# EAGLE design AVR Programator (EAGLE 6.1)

## Sheet 1 of 3: Atmel programmer
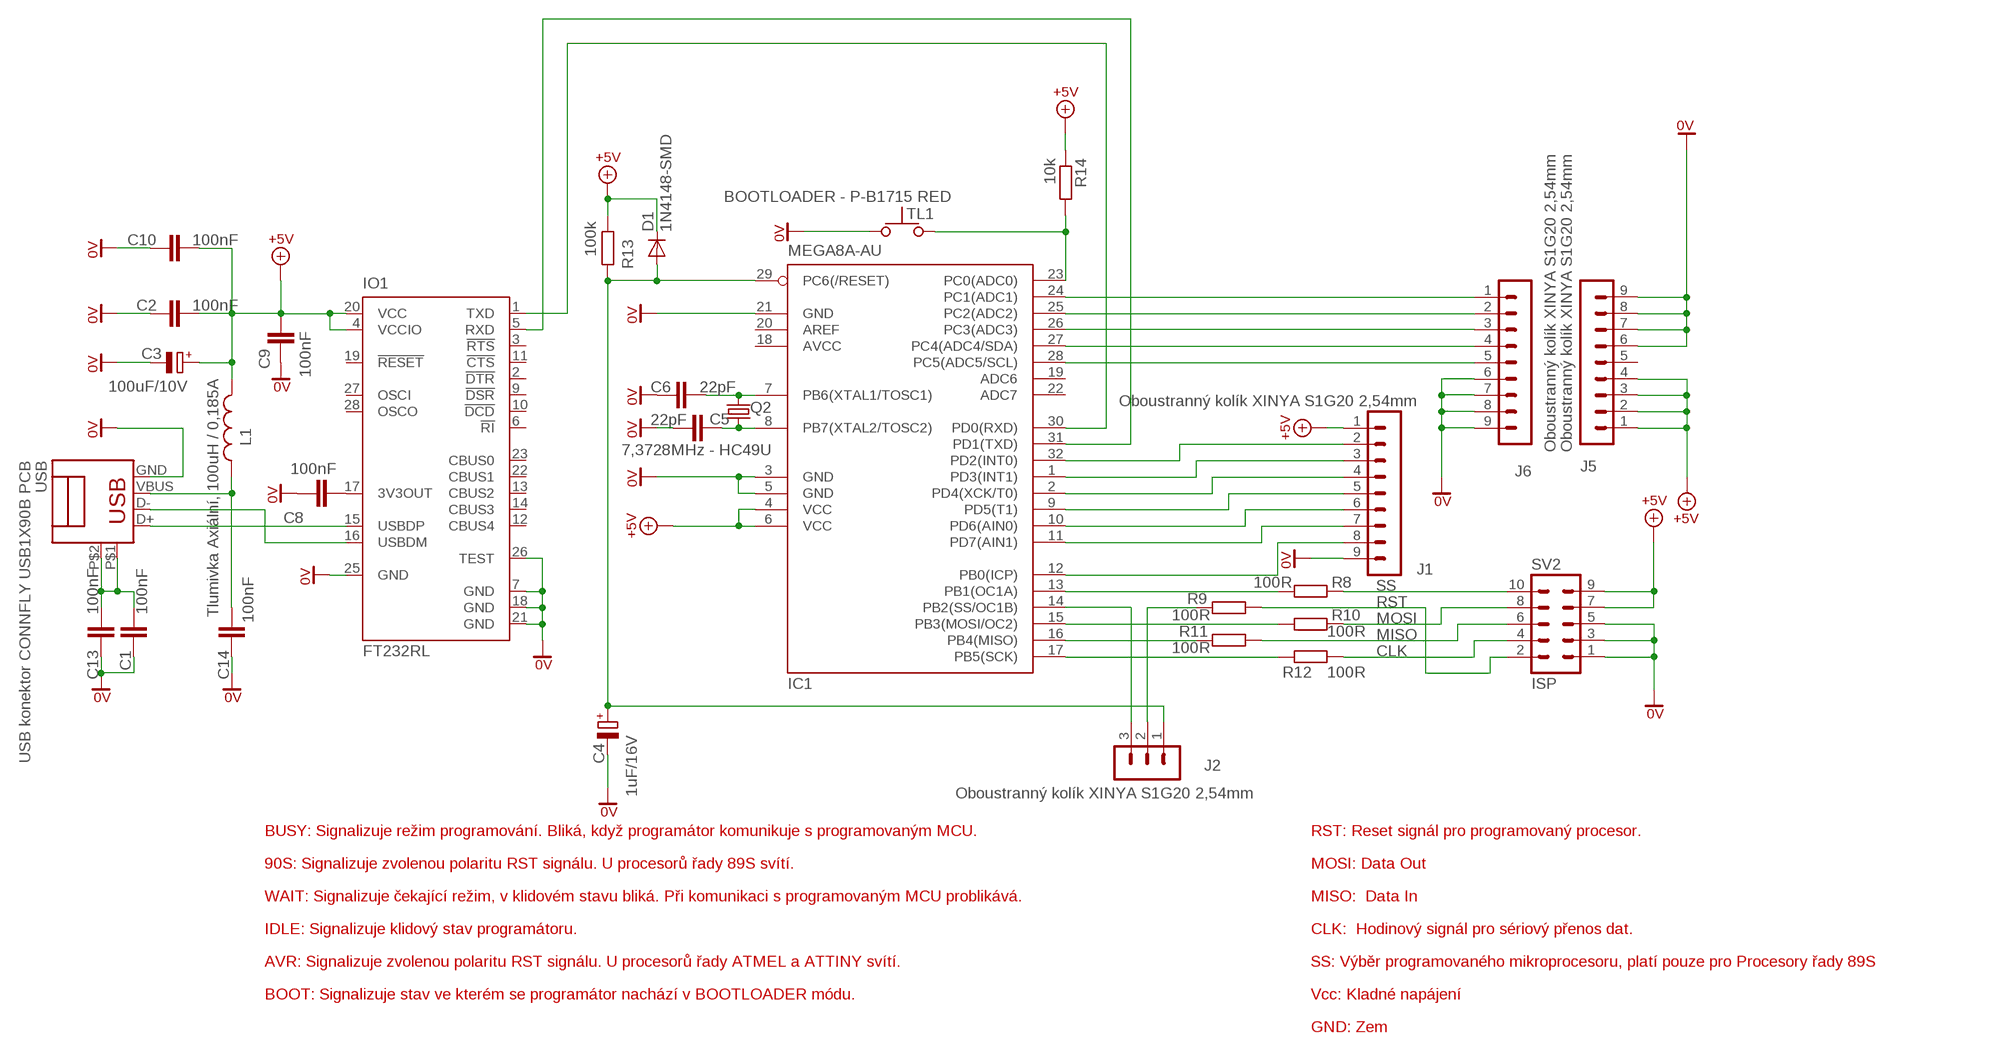
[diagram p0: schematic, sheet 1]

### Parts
C1  100nF  C-EU025-024X044  [C025-024X044]
C2  100nF  C-EU025-024X044  [C025-024X044]
C3  100uF/10V  CPOL-EUSMCE  [SMC_E]
C4  1uF/16V  CPOL-EUSMCC  [SMC_C]
C5  22pF  C-EUC1206K  [C1206K]
C6  22pF  C-EUC1206K  [C1206K]
C8  100nF  C-EU025-024X044  [C025-024X044]
C9  100nF  C-EU025-024X044  [C025-024X044]
C10  100nF  C-EUC1206  [C1206]
C13  100nF  C-EU025-024X044  [C025-024X044]
C14  100nF  C-EU025-024X044  [C025-024X044]
D1  1N4148-SMD  [SOD80C]
IC1  MEGA8A-AU  MEGA8-AI  [TQFP32-08]
IO1  FT232RL  [SSOP28]
J1  Oboustranný kolík XINYA S1G20 2,54mm  MA09-1  [MA09-1]
J2  Oboustranný kolík XINYA S1G20 2,54mm  MA03-1  [MA03-1]
J5  Oboustranný kolík XINYA S1G20 2,54mm  MA09-1  [MA09-1]
J6  Oboustranný kolík XINYA S1G20 2,54mm  MA09-1  [MA09-1]
L1  Tlumivka Axiální, 100uH / 0,185A  L-US0207/10  [0207/10]
Q2  7,3728MHz - HC49U  CRYSTALSMD  [HC49UP]
R8  100R  R-EU_M1206  [M1206]
R9  100R  R-EU_M1206  [M1206]
R10  100R  R-EU_M1206  [M1206]
R11  100R  R-EU_M1206  [M1206]
R12  100R  R-EU_M1206  [M1206]
R13  100k  R-EU_0204/7  [0204/7]
R14  10k  R-EU_0204/7  [0204/7]
SV2  ISP  MLW10  [ML10]
TL1  BOOTLOADER - P-B1715 RED  TLACITKO  [H]
USB  USB konektor CONNFLY USB1X90B PCB  USB4  [USB-B-H]

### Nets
0V: C1.1 C2.1 C3.- C4.- C5.2 C6.2 C8.1 C9.2 C10.1 C13.1 C14.1 IC1.3(GND) IC1.5(GND) IC1.21(GND) IO1.7(GND) IO1.18(GND) IO1.21(GND) IO1.25(GND) IO1.26(TEST) J1.9 J5.6 J5.7 J5.8 J5.9 J6.6 J6.7 J6.8 J6.9 SV2.1 SV2.3 SV2.5 TL1.P$1 USB.GND
+5V: C2.2 C3.+ C9.1 C10.2 D1.C IC1.4(VCC) IC1.6(VCC) IO1.4(VCCIO) IO1.20(VCC) J1.1 J5.1 J5.2 J5.3 J5.4 L1.2 R13.2 R14.1 SV2.7 SV2.9
CLK: R12.2 SV2.4
MISO: R11.2 SV2.6
MOSI: R10.2 SV2.8
N$1: C14.2 L1.1 USB.VBUS
N$3: C4.+ D1.A IC1.29(PC6(/RESET)) J2.1 R13.1
N$4: IO1.15(USBDP) USB.D+
N$5: IO1.16(USBDM) USB.D-
N$6: IC1.30(PD0(RXD)) IO1.1(TXD)
N$7: IC1.31(PD1(TXD)) IO1.5(RXD)
N$8: C6.1 IC1.7(PB6(XTAL1/TOSC1)) Q2.2
N$9: C5.1 IC1.8(PB7(XTAL2/TOSC2)) Q2.1
N$10: IC1.14(PB2(SS/OC1B)) J2.3
N$11: IC1.12(PB0(ICP)) J1.8
N$12: IC1.11(PD7(AIN1)) J1.7
N$13: IC1.10(PD6(AIN0)) J1.6
N$14: IC1.9(PD5(T1)) J1.5
N$15: IC1.2(PD4(XCK/T0)) J1.4
N$16: IC1.1(PD3(INT1)) J1.3
N$17: IC1.32(PD2(INT0)) J1.2
N$18: IC1.23(PC0(ADC0)) R14.2 TL1.P$2
N$19: IC1.24(PC1(ADC1)) J6.1
N$21: IC1.25(PC2(ADC2)) J6.2
N$23: IC1.26(PC3(ADC3)) J6.3
N$27: IC1.27(PC4(ADC4/SDA)) J6.4
N$30: IC1.13(PB1(OC1A)) R8.1
N$31: IC1.28(PC5(ADC5/SCL)) J6.5
N$33: IC1.15(PB3(MOSI/OC2)) R10.1
N$38: IC1.17(PB5(SCK)) R12.1
N$39: IC1.16(PB4(MISO)) R11.1
N$40: J2.2 R9.1
N$41: C8.2 IO1.17(3V3OUT)
N$45: C1.2 C13.2 USB.P$1(SHILED) USB.P$2(SHILED)
RST: R9.2 SV2.2
SS: R8.2 SV2.10
Unconnected: IC1.19(ADC6) IC1.20(AREF) IC1.22(ADC7) IO1.2(!DTR) IO1.3(!RTS) IO1.6(!RI) IO1.9(!DSR) IO1.10(!DCD) IO1.11(!CTS) IO1.12(CBUS4) IO1.13(CBUS2) IO1.14(CBUS3) IO1.19(!RESET) IO1.22(CBUS1) IO1.23(CBUS0) IO1.27(OSCI) IO1.28(OSCO) J5.5

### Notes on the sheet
- BUSY: Signalizuje režim programování. Bliká, když programátor komunikuje s programovaným MCU. | RST: Reset signál pro programovaný procesor.
- 90S: Signalizuje zvolenou polaritu RST signálu. U procesorů řady 89S svítí. | MOSI: Data Out
- WAIT: Signalizuje čekající režim, v klidovém stavu bliká. Při komunikaci s programovaným MCU problikává. | MISO:  Data In
- IDLE: Signalizuje klidový stav programátoru. | CLK:  Hodinový signál pro sériový přenos dat.
- AVR: Signalizuje zvolenou polaritu RST signálu. U procesorů řady ATMEL a ATTINY svítí. | SS: Výběr programovaného mikroprocesoru, platí pouze pro Procesory řady 89S
- BOOT: Signalizuje stav ve kterém se programátor nachází v BOOTLOADER módu. | Vcc: Kladné napájení
- GND: Zem

## Sheet 2 of 3: LED driver
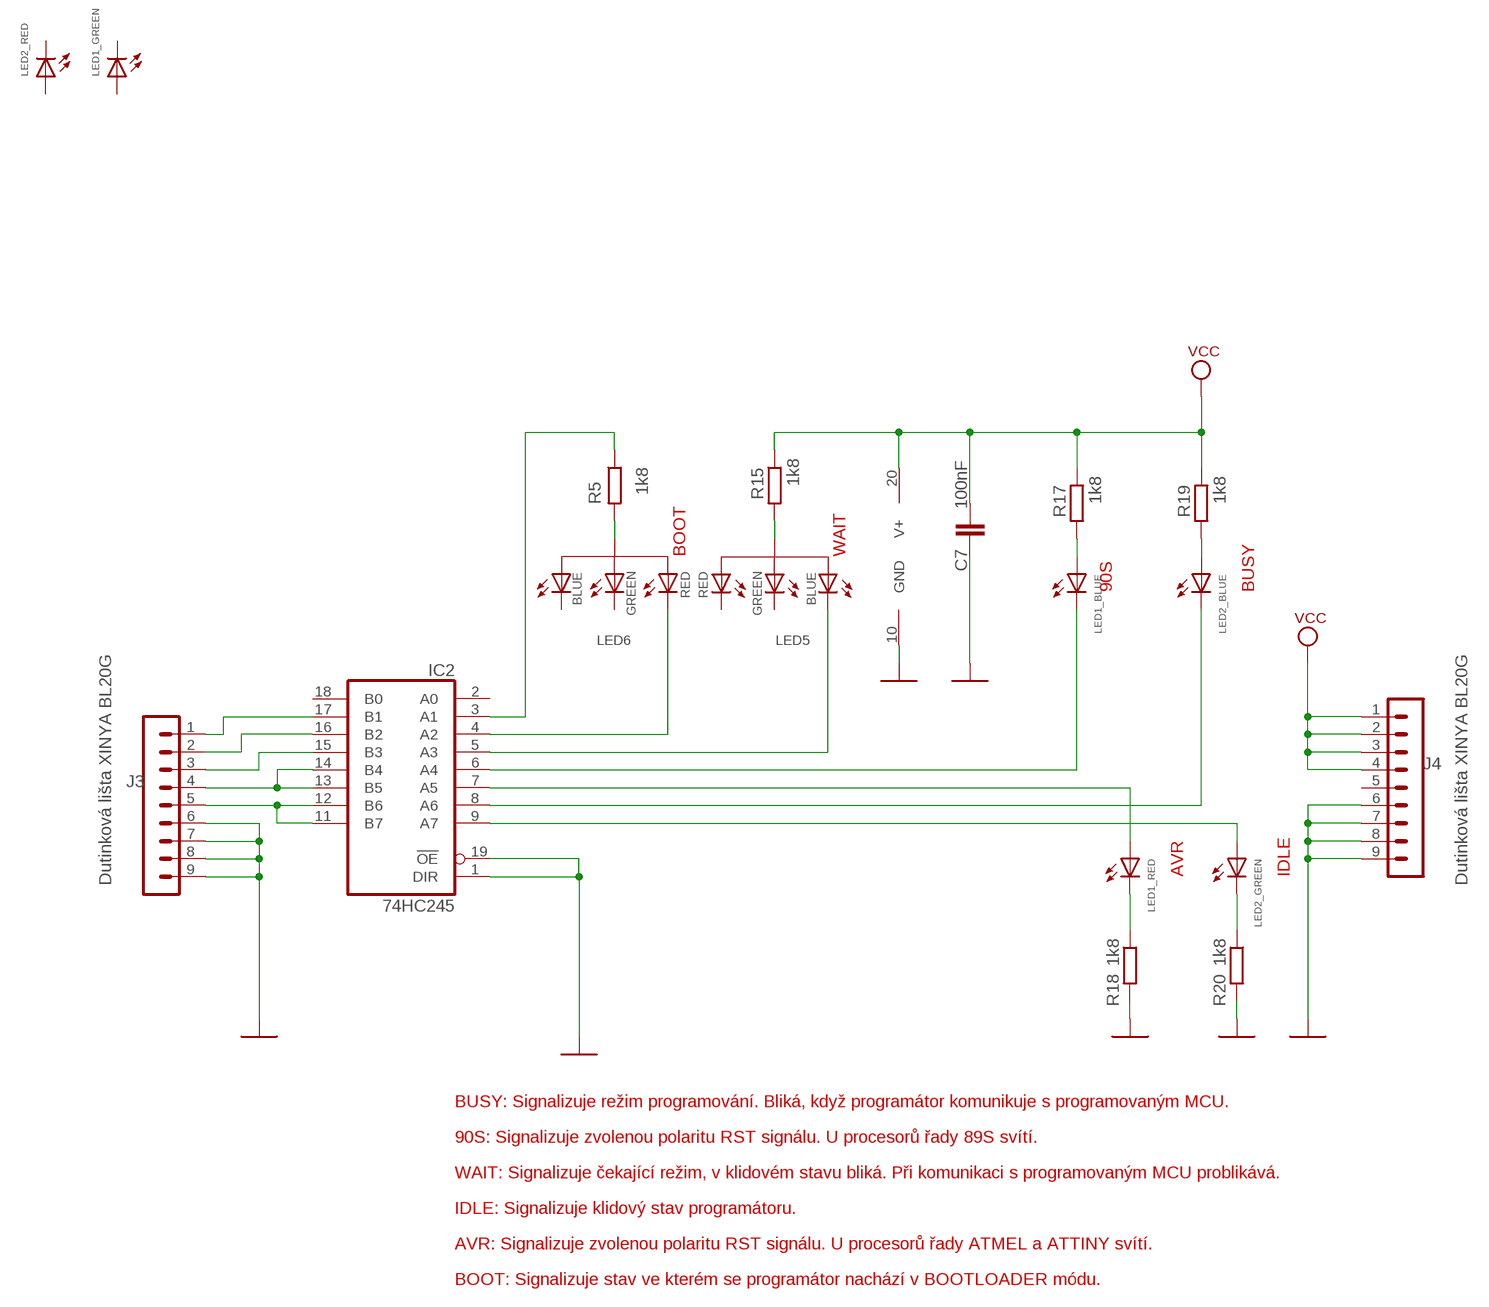
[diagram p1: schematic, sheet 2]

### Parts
C7  100nF  C-EU025-024X044  [C025-024X044]
IC2  74HC245  IC_BUFF_74LVC245A-SSOP20  [SSOP-20]
J3  Dutinková lišta XINYA BL20G  MA09-1  [MA09-1]
J4  Dutinková lišta XINYA BL20G  MA09-1  [MA09-1]
LED1  LED_PLCC6  [LED_PLCC6]
LED2  LED_PLCC6  [LED_PLCC6]
LED5  LED_PLCC4  [LED_PLCC4]
LED6  LED_PLCC4  [LED_PLCC4]
R5  1k8  R-EU_0204/7  [0204/7]
R15  1k8  R-EU_0204/7  [0204/7]
R17  1k8  R-EU_0204/7  [0204/7]
R18  1k8  R-EU_0204/7  [0204/7]
R19  1k8  R-EU_0204/7  [0204/7]
R20  1k8  R-EU_0204/7  [0204/7]

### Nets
GND: C7.1 IC2.1(DIR) IC2.10(GND) IC2.19(!OE) J3.6 J3.7 J3.8 J3.9 J4.6 J4.7 J4.8 J4.9 R18.2 R20.2
N$2: IC2.15(B3) J3.3
N$20: IC2.5(A3) LED5.B
N$22: IC2.4(A2) LED6.R
N$24: LED6.A R5.2
N$25: IC2.16(B2) J3.2
N$26: IC2.17(B1) J3.1
N$28: LED1.R(-K) R18.1
N$29: LED5.A R15.2
N$51: LED1.+B(+A) R17.2
N$53: LED2.+B(+A) R19.2
N$54: LED2.G(-K) R20.1
N$55: IC2.3(A1) R5.1
N$58: IC2.13(B5) IC2.14(B4) J3.4
N$59: IC2.11(B7) IC2.12(B6) J3.5
N$60: IC2.6(A4) LED1.B(-K)
N$61: IC2.7(A5) LED1.+R(+A)
N$62: IC2.9(A7) LED2.+G(+A)
N$63: IC2.8(A6) LED2.B(-K)
V+: C7.2 IC2.20(V+) J4.1 J4.2 J4.3 J4.4 R15.1 R17.1 R19.1 ; supply symbol labelled VCC
Unconnected: IC2.2(A0) IC2.18(B0) J4.5 LED1.+G(+A) LED1.G(-K) LED2.+R(+A) LED2.R(-K) LED5.G LED5.R LED6.B LED6.G

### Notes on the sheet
- BOOT | WAIT
- 90S | BUSY
- AVR | IDLE
- BUSY: Signalizuje režim programování. Bliká, když programátor komunikuje s programovaným MCU.
- 90S: Signalizuje zvolenou polaritu RST signálu. U procesorů řady 89S svítí.
- WAIT: Signalizuje čekající režim, v klidovém stavu bliká. Při komunikaci s programovaným MCU problikává.
- IDLE: Signalizuje klidový stav programátoru.
- AVR: Signalizuje zvolenou polaritu RST signálu. U procesorů řady ATMEL a ATTINY svítí.
- BOOT: Signalizuje stav ve kterém se programátor nachází v BOOTLOADER módu.

## Sheet 3 of 3: Kabel k BeeProg
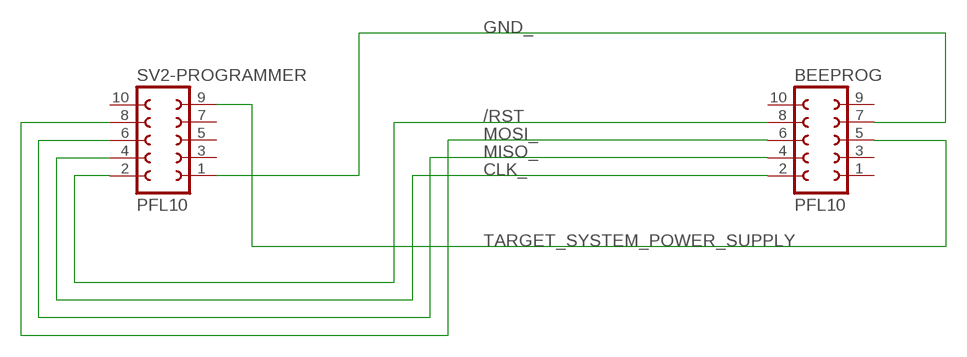
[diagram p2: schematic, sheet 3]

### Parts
BEEPROG  PFL10  [ML10]
SV2-PROGRAMMER  PFL10  [ML10]

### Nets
/RST: BEEPROG.8 SV2-PROGRAMMER.2
CLK_: BEEPROG.2 SV2-PROGRAMMER.4
GND_: BEEPROG.7 SV2-PROGRAMMER.1
MISO_: BEEPROG.4 SV2-PROGRAMMER.6
MOSI_: BEEPROG.6 SV2-PROGRAMMER.8
TARGET_SYSTEM_POWER_SUPPLY: BEEPROG.5 SV2-PROGRAMMER.9
Unconnected: BEEPROG.1 BEEPROG.3 BEEPROG.9 BEEPROG.10 SV2-PROGRAMMER.3 SV2-PROGRAMMER.5 SV2-PROGRAMMER.7 SV2-PROGRAMMER.10

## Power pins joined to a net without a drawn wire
AVCC: IC1.18(AVCC)

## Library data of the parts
BEEPROG SV2-PROGRAMMER = con-ml:PFL10
C1 C2 C5-C10 C13 C14 = rcl:C-EU: CAPACITOR, European symbol
C3 C4 = resistor:CPOL-EU: POLARIZED CAPACITOR, European symbol
D1 = #hacesoft:1N4148: DIODE
IC1 = atmel:MEGA8: MICROCONTROLLER 8 Kbytes FLASH, 1 kbytes SRAM, 512 bytes EEPROM, USART, 6-channel 10 bit ADC, 2-channel 8 bit ADC Pin compatible with Atmega48, ATMega88, ATMega168 Source: avr.lbr; MPN: ATMEGA8-16AU; OC_FARNELL: 9171371; OC_NEWARK: 73M8863
IC2 = xxx:IC_BUFF_74LVC245A: Octal Bus transceiver with 3-state, 3.3V supply
IO1 = ftdichip:FT232R: Source: http://www.ftdichip.com/Documents/DataSheets/DS_FT232R_v104.pdf
J1 J3-J6 = con-lstb:MA09-1: PIN HEADER
J2 = con-lstb:MA03-1: PIN HEADER
L1 = rcl:L-US: INDUCTOR, American symbol
LED1 LED2 = #hacesoft:LED_PLCC6
LED5 LED6 = #hacesoft:LED_PLCC4
Q2 = SparkFun-3-2-07:CRYSTAL: Crystals
R5 R8-R15 R17-R20 = rcl:R-EU_: RESISTOR, European symbol
SV2 = #hacesoft:MLW10: HARTING
TL1 = #hacesoft:TLACITKO
USB = #hacesoft:USB: USB Connectors

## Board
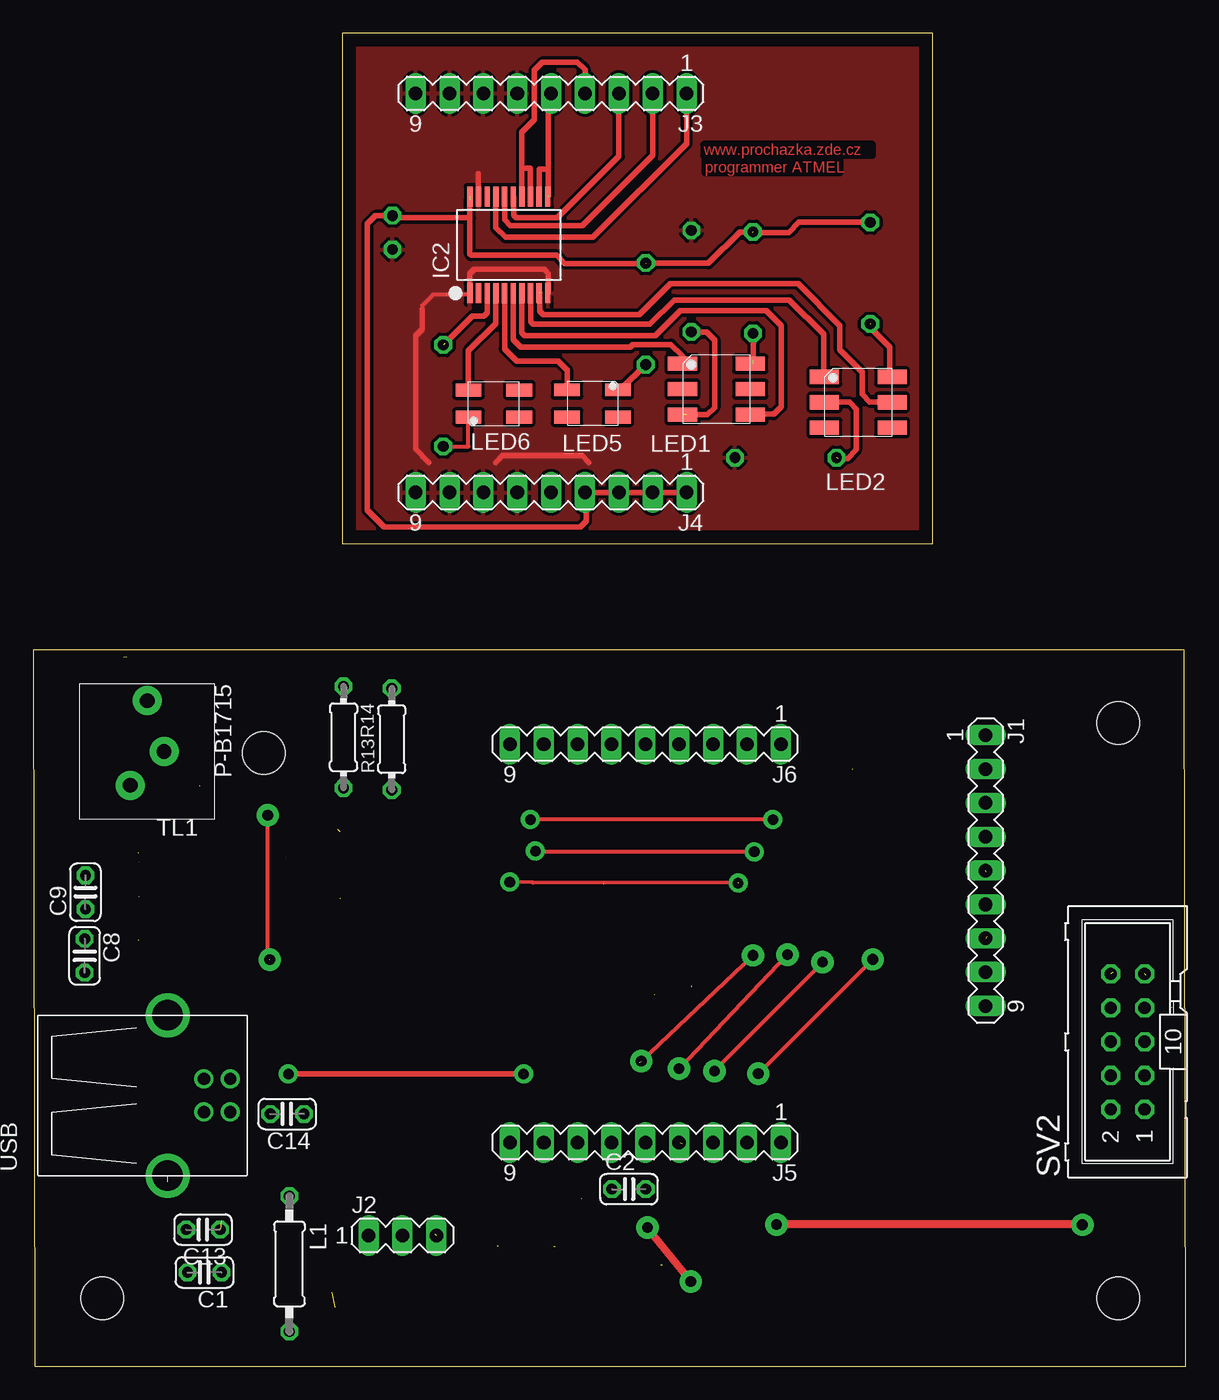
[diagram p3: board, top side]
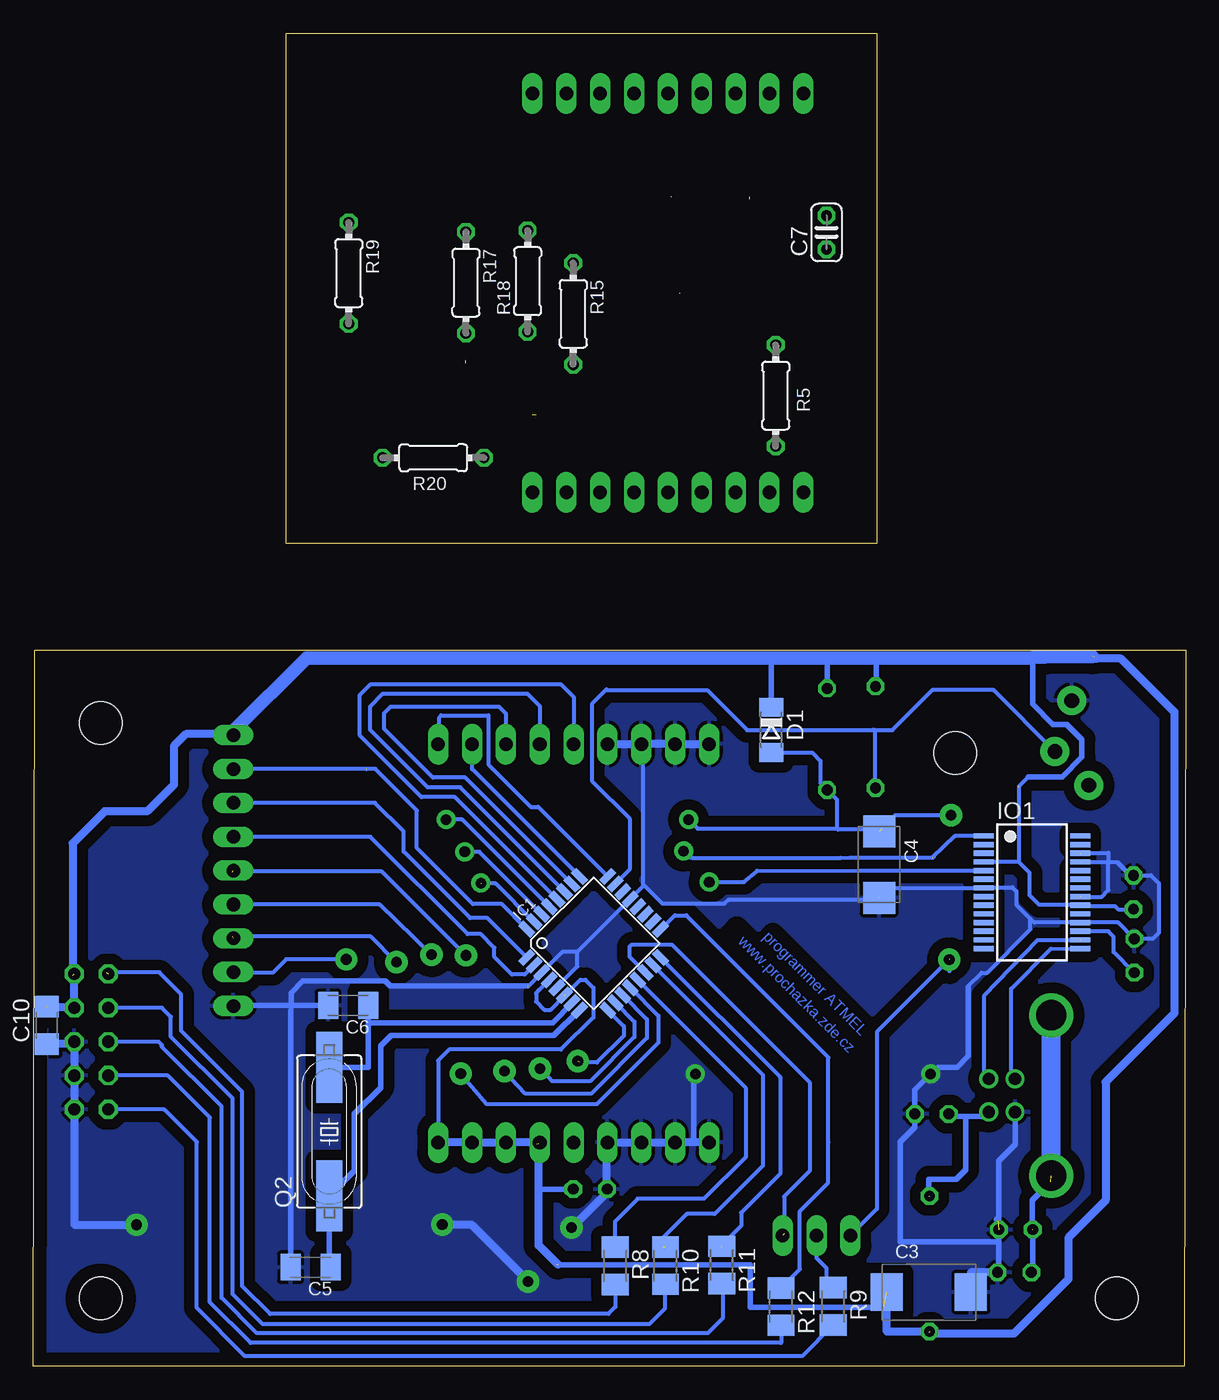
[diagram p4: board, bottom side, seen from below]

Size 86.44 x 100.02 mm. Coordinates in mm from the lower left corner, seen from the top.
Outline: 0.1,0 86.44,0 86.34,53.74 0,53.74 0.1,0
Outline: 23.17,61.72 67.47,61.72 67.47,100.02 23.17,100.02 23.17,61.72
Copper layers (1*16): Top 0.035mm / dielectric 1.5mm / Bottom 0.035mm
Design rules: minimum track width 10mil, minimum drill 24mil, track to track 8mil, track to pad 8mil, pad to pad 8mil, via to via 8mil, smd to smd 8mil, copper to edge 40mil, drill to drill 8mil, minimum pad ring 10mil, minimum via ring 8mil, stop-mask expansion 4mil, vias tented up to drill 0mil, thermal gap 10mil
Holes 3.2 mm at 5.18,5.08 81.38,5.08 81.38,48.26 17.3,46.03

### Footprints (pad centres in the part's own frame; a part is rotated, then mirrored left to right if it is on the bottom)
ML10 = drill 1.016 octagon: 1 -5.08,-1.27 | drill 1.016: 2 -5.08,1.27; 3 -2.54,-1.27; 4 -2.54,1.27; 5 0,-1.27; 6 0,1.27; 7 2.54,-1.27; 8 2.54,1.27; 9 5.08,-1.27; 10 5.08,1.27
C025-024X044 = drill 0.813 octagon: 1 -1.27,0; 2 1.27,0
SMC_E = smd 2.4 x 2.8: + -3.15,0; - 3.15,0
SMC_C = smd 2.4 x 2.4: + -2.5,0; - 2.5,0
C1206K = smd 1.5 x 2: 1 -1.5,0; 2 1.5,0
C1206 = smd 1.6 x 1.8: 1 -1.4,0; 2 1.4,0
SOD80C = smd 1.4 x 1.8: A 1.7,0; C -1.7,0
TQFP32-08 = smd 1.27 x 0.559: 1 -4.293,2.8; 2 -4.293,2; 3 -4.293,1.2; 4 -4.293,0.4; 5 -4.293,-0.4; 6 -4.293,-1.2; 7 -4.293,-2; 8 -4.293,-2.8; 17 4.293,-2.8; 18 4.293,-2; 19 4.293,-1.2; 20 4.293,-0.4; 21 4.293,0.4; 22 4.293,1.2; 23 4.293,2; 24 4.293,2.8 | smd 0.559 x 1.27: 9 -2.8,-4.293; 10 -2,-4.293; 11 -1.2,-4.293; 12 -0.4,-4.293; 13 0.4,-4.293; 14 1.2,-4.293; 15 2,-4.293; 16 2.8,-4.293; 25 2.8,4.293; 26 2,4.293; 27 1.2,4.293; 28 0.4,4.293; 29 -0.4,4.293; 30 -1.2,4.293; 31 -2,4.293; 32 -2.8,4.293
SSOP-20 = smd 0.4 x 1.5: 1 -2.925,-3.625; 2 -2.275,-3.625; 3 -1.625,-3.625; 4 -0.975,-3.625; 5 -0.325,-3.625; 6 0.325,-3.625; 7 0.975,-3.625; 8 1.625,-3.625; 9 2.275,-3.625; 10 2.925,-3.625; 11 2.925,3.625; 12 2.275,3.625; 13 1.625,3.625; 14 0.975,3.625; 15 0.325,3.625; 16 -0.325,3.625; 17 -0.975,3.625; 18 -1.625,3.625; 19 -2.275,3.625; 20 -2.925,3.625
SSOP28 = smd 0.4 x 1.5: 1 -4.225,-3.625; 2 -3.575,-3.625; 3 -2.925,-3.625; 4 -2.275,-3.625; 5 -1.625,-3.625; 6 -0.975,-3.625; 7 -0.325,-3.625; 8 0.325,-3.625; 9 0.975,-3.625; 10 1.625,-3.625; 11 2.275,-3.625; 12 2.925,-3.625; 13 3.575,-3.625; 14 4.225,-3.625; 15 4.225,3.625; 16 3.575,3.625; 17 2.925,3.625; 18 2.275,3.625; 19 1.625,3.625; 20 0.975,3.625; 21 0.325,3.625; 22 -0.325,3.625; 23 -0.975,3.625; 24 -1.625,3.625; 25 -2.275,3.625; 26 -2.925,3.625; 27 -3.575,3.625; 28 -4.225,3.625
MA09-1 = drill 1.016 long: 1 -10.16,0; 2 -7.62,0; 3 -5.08,0; 4 -2.54,0; 5 0,0; 6 2.54,0; 7 5.08,0; 8 7.62,0; 9 10.16,0
MA03-1 = drill 1.016 long: 1 -2.54,0; 2 0,0; 3 2.54,0
0207/10 = drill 0.813 octagon: 1 -5.08,0; 2 5.08,0
LED_PLCC6 = smd 2.184 x 1.067: +B 2.61,1.855; +G 2.61,-0.05; +R 2.61,-1.955; B -2.47,1.855; G -2.47,-0.05; R -2.47,-1.955
LED_PLCC4 = smd 1.93 x 0.965: A 1.83,0.785; B -1.98,0.785; G -1.98,-1.247; R 1.83,-1.247
HC49UP = smd 5.334 x 1.93: 1 -4.826,0; 2 4.826,0
0204/7 = drill 0.813 octagon: 1 -3.81,0; 2 3.81,0
M1206 = smd 1.6 x 2: 1 -1.4,0; 2 1.4,0
ML10' = drill 0.914 octagon: 1 -5.08,-1.27; 2 -5.08,1.27; 3 -2.54,-1.27; 4 -2.54,1.27; 5 0,-1.27; 6 0,1.27; 7 2.54,-1.27; 8 2.54,1.27; 9 5.08,-1.27; 10 5.08,1.27
H = drill 1.1 pad 2.184: P$1 1.27,-3.81; P$2 0,0; P$11 2.54,2.54
USB-B-H = drill 0.914: D+ 0,1.25; D- 1.981,1.25; GND 0,-1.25; VBUS 1.981,-1.25 | drill 2.286: P$1 -2.718,-6.02; P$2 -2.718,6.02

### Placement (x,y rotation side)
BEEPROG  not placed on the board
C1  12.84,7.04 180 top
C2  44.67,13.29 0 top
C3  19.26,5.56 0 bottom
C4  23,37.64 270 bottom
C5  65.64,7.43 180 bottom
C6  62.83,27.07 180 bottom
C7  26.94,85.07 90 bottom
C8  3.85,30.8 270 top
C9  3.91,35.56 90 top
C10  85.43,25.57 90 bottom
C13  12.74,10.25 180 top
C14  19.04,18.93 180 top
D1  31.07,47.75 270 bottom
IC1  44.41,31.73 45 bottom
IC2  35.67,84.14 0 top
IO1  11.53,35.56 270 bottom
J1  71.44,37.19 270 top
J2  27.69,9.81 0 top
J3  38.84,95.51 180 top
J4  38.84,65.57 180 top
J5  45.91,16.79 180 top
J6  45.91,46.68 180 top
L1  19.21,7.68 270 top
LED1  51.17,73.37 0 top
LED2  61.81,72.38 0 top
LED5  42.02,72.48 0 top
LED6  34.47,72.01 180 top
Q2  64.24,17.6 90 bottom
R5  30.75,72.83 270 bottom
R8  42.79,7.53 270 bottom
R9  26.43,4.49 270 bottom
R10  39.03,7.55 270 bottom
R11  34.8,7.59 270 bottom
R12  30.35,4.47 270 bottom
R13  26.89,47.05 90 top
R14  23.27,47.2 270 top
R15  45.94,78.97 270 bottom
R17  53.99,81.31 270 bottom
R18  49.36,81.42 90 bottom
R19  62.78,82.02 270 bottom
R20  56.44,68.17 0 bottom
SV2  ISP  [ML10']  82.09,24.35 90 top
SV2-PROGRAMMER  not placed on the board
TL1  9.81,46.13 180 top
USB  12.8,20.32 0 top

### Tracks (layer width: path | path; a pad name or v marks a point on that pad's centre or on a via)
0V  (via drill 0.8 pad 1.42, 0.8 pad 1.68)  (7 unrouted)
  Top 0.406: v19.13,21.92 v36.79,21.92
  Top 0.61: v78.69,10.61 78.69,10.63 v55.76,10.63 | v49.32,6.36 v46.06,10.39
  Bottom 0.305: 5.8,37.83 5.2,37.83 | 5.2,37.83 5.1,37.83 4.1,36.83 | 7.86,38.53 5.8,38.53 5.8,37.83 | IO1.25 5.8,37.83 | 5.2,37.83 4.2,36.83 2.6,36.83 2,36.23 2,32.53 2.46,32.07 C8.1 5.06,33.28 IO1.18 11.36,33.28 11.65,33.58 | IO1.21 6.3,35.23 5.8,35.73 5.8,37.83 | USB.GND 13.09,18.78 12.99,18.78 | 15.11,35.93 13,35.93 12.7,35.63 12.7,34.63 11.65,33.58 | 16.3,28.53 15.3,29.53 14.9,29.53 11.65,32.78 11.65,33.58 | 45.63,31.08 IC1.21 40.67,36.04 40.67,46.13 40.83,46.29 J6.7 | 45.63,31.08 46.76,31.08 IC1.3 49.36,28.48 | IC1.5 47.16,28.45 45.63,29.99 45.63,31.08 | 67.11,26.8 67.11,27.13 64.39,27.13 C6.2 | IO1.7 15.18,35.86 22.27,35.86 23.03,35.1 | 40.7,36.15 39.26,34.71 34.6,34.71 34.29,35.02 23.03,35.02 22.28,35.77 22.23,35.77
  Bottom 0.406: C6.2 71.4,27.07 J1.9 | C5.2 67.14,26.7 | 67.11,27.13 67.11,28.03 66.23,28.91 60.03,28.91 59.66,28.54 49.36,28.54 | 16.31,28.45 16.31,23.27 17.15,22.43 18.6,22.43 20.31,20.72 C14.1 20.31,17.92 21.4,16.83 21.4,9.33 14.11,9.33 | J5.9 arc90 J5.9 | C2.1 43.37,13.29 J5.6 | C1.1 14.01,7.14 C13.1 14.01,15.42 12.8,16.63 USB.GND | 14.2,11.03 arc90 14.1,10.93 | v36.78,21.92 36.9,21.92 36.9,16.78
  Bottom 0.61: J6.6 J6.7 J6.8 J6.9 | J5.6 J5.7 J5.8 J5.9 | v78.69,10.61 83.36,10.61 SV2.1 SV2.3 SV2.5 83.36,24.17 C10.1 | v55.76,10.63 53.59,10.63 v49.32,6.36 | v46.06,10.39 43.4,13.05 43.4,13.45 43.42,13.45 43.44,13.47 43.44,16.84 | C1.1 16.11,7.04 C3.-
  pour Bottom (isolate 0.813): 0.01,53.8 86.65,53.8 86.65,-0.1 -0.13,-0.42
+5V  (9 unrouted)
  Bottom 0.305: C9.1 5.06,34.29 5.3,34.53 7.85,34.53 IO1.20 7.95,34.63 11,34.63 11.7,35.33 11.7,37.03 12.5,37.83 | 12.5,37.83 IO1.4 | IC1.4 48.51,28.2 48.53,28.2 48.72,28.01 48.72,27.37 48.1,26.75 47.64,26.75 46.62,27.77 46.62,27.87 46.59,27.87 46.55,27.91 46.49,27.91 45.41,28.99 45.03,28.99 44.43,28.39 44.43,26.19 | 44.43,26.19 44.43,26.17 | 48.47,16.48 48.67,16.68 48.67,16.8 | 12.5,43.48 12.5,37.83 | 44.43,26.19 46.86,23.76 55.24,23.76 56.07,22.93 J5.1 | 11.8,44.23 12.5,43.53
  Bottom 0.406: C2.2 48.53,13.29 48.53,13.45 | D1.C 31.07,53 | 31.07,53 31.1,53.03 | R13.2 26.89,53.15 | 26.89,53.15 26.9,53.16 | 26.89,53.15 23.32,53.15 23.2,53.03 23.2,51.08 R14.1 | 26.89,53.15 30.92,53.15 31.07,53 | 22.64,4.42 32.67,4.42 32.67,7.62 47.18,7.62 | 11.8,44.23 9.26,44.23 7.79,45.7 7.79,47.03 8.93,48.17 9.95,48.17 11.48,49.7 11.48,53.17
  Bottom 0.61: J5.1 J5.2 J5.3 J5.4 48.53,16.71 48.53,13.45 48.53,9.07 47.08,7.62 | 71.47,47.38 J1.1 71.52,47.43 75,47.43 75.9,46.53 75.9,43.63 77.9,41.63 81.1,41.63 83.5,39.23 83.5,29.33 | SV2.9 SV2.7 83.36,26.94 85.38,26.94 | 19.27,2.49 19.27,2.44 12.89,2.44 8.8,6.53 8.8,9.63 6,12.43 6,21.33 0.85,26.48 0.85,49.1 4.85,53.1 6.69,53.1 6.8,53.21 | L1.2 22.41,2.6 C3.+
  Bottom 1.016: 7.02,53.25 10.57,53.2 11.48,53.17 11.73,53.16 26.9,53.16 65.93,53.16 71.44,47.65 J1.1
/RST  (1 unrouted)
CLK
  Bottom 0.305: R12.2 30.35,1.74 70.14,1.74 73.2,4.8 73.2,18.66 76.35,21.81 SV2.4
CLK_  (1 unrouted)
GND
  Top 0.305: IC2.1 32.65,80.42 29.99,80.42 29.17,79.6 29.17,79.32
  Top 0.406: 41.67,67.82 41.17,68.32 35.17,68.32 34.67,67.82 | 29.67,67.82 28.67,68.82 28.67,77.32 29.17,77.82 29.17,79.32 | IC2.19 33.38,87.78 33.38,89.48 | IC2.10 38.63,80.55 38.63,81.99 38.31,82.31 33.08,82.31 32.75,81.97 IC2.1
  pour Top (isolate 0.254): 67.72,100.06 23.09,100.06 23.09,61.69 67.66,61.69 67.66,100.03
GND_  (1 unrouted)
MISO
  Bottom 0.305: R11.2 34.74,6.13 34.74,3.58 35.84,2.48 69.67,2.48 72.31,5.12 72.31,19.48 76.79,23.96 76.79,24.1 77.04,24.35 SV2.6
MISO_  (1 unrouted)
MOSI
  Bottom 0.305: R10.2 39.07,6.11 39.07,4.31 40.23,3.15 69.23,3.15 71.49,5.41 71.49,20.1 76.12,24.73 76.12,26.23 76.79,26.9 SV2.8
MOSI_  (1 unrouted)
N$1  (1 unrouted)
  Bottom 0.406: USB.VBUS 15.12,18.73 16.5,18.73 | 16.5,18.73 17.77,18.73 | 16.5,18.73 16.5,14.73 17.2,14.03 19.27,14.03 19.27,12.78 | 17.9,18.73 17.77,18.73 | 17.77,18.73 C14.2
N$2
  Top 0.406: IC2.15 36.02,87.74 36.02,86.37 36.22,86.17 39.3,86.17 43.92,90.79 J3.3
N$3  (via drill 0.8 pad 1.42, 0.8 pad 1.68)  (2 unrouted)
  Top 0.305: v17.73,30.51 17.59,30.45 v17.59,41.34 | v55.48,41.02 v37.29,41.02
  Bottom 0.305: C4.+ 23.12,40.26 26.08,40.26 26.15,40.33 26.15,40.34 | 17.79,30.51 v17.73,30.51 23.16,25.08 23.16,11.8 J2.1 | IC1.29 54.27,41.02 v55.48,41.02 | v37.29,41.02 36.61,40.34 26.15,40.34 | v17.59,41.34 21.79,41.34 22.8,40.33 | D1.A 28.02,46.05 27.4,45.43 27.4,43.75 R13.1 26.15,42.5 26.15,40.34 | 17.7,29.63 17.7,30.53
N$4
  Bottom 0.305: USB.D+ 13.1,21.87 13.1,28.33 10.1,31.33 IO1.15
N$5  (1 unrouted)
  Bottom 0.305: USB.D- 15.1,21.57 15.1,27.83 11.1,31.98 7.87,31.98
N$6  (via drill 0.8 pad 1.42)  (1 unrouted)
  Top 0.305: v54.08,38.6 37.71,38.6 v37.66,38.65
  Bottom 0.305: IO1.1 17.3,39.78 18.99,38.19 | IC1.30 52.98,38.6 v54.08,38.6 | v37.66,38.65 37.66,38.33 36.98,38.15 25.89,38.15 25.17,38.17 18.97,38.17 18.89,38.24
N$7  (via drill 0.8 pad 1.42)  (1 unrouted)
  Top 0.305: v52.87,36.25 37.47,36.3 v35.74,36.33
  Bottom 0.305: IC1.31 48.9,33.35 51.77,36.22 52.84,36.22 | v35.74,36.33 33.13,36.33 32.14,37.18 24.51,37.18 IO1.5
N$8
  Bottom 0.406: Q2.2 61.33,22.43 61.33,25.62 | 61.33,25.62 C6.1 | IC1.7 46.03,27.21 47.46,25.78 61.17,25.78 61.33,25.62
N$9
  Bottom 0.406: C5.1 64.24,7.53 Q2.1 62.36,14.65 62.36,18.92 60.39,20.89 60.39,24.02 59.58,24.83 47.39,24.83 45.5,26.72 IC1.8
N$10  (1 unrouted)
  Bottom 0.305: IC1.14 41.7,30.72 41.7,31.49 41.54,31.65 38.55,31.65 28.21,21.31 28.21,14.65 30.12,12.74 30.12,9.93
N$11  (via drill 0.8 pad 1.68)
  Top 0.305: v54.38,21.95 v54.39,21.95 v62.97,30.53
  Bottom 0.305: IC1.12 39.55,26.3 39.55,24.27 44.16,19.66 52.44,19.66 v54.38,21.95 | v62.97,30.53 67.48,30.53 68.49,29.52 71.39,29.52 J1.8
N$12  (via drill 0.8 pad 1.68)  (1 unrouted)
  Top 0.305: v51.1,22.14 51.1,22.21 v59.2,30.31
  Bottom 0.305: IC1.11 40.42,26.04 40.42,24.62 44.59,20.45 49.52,20.45 v51.1,22.14 | v59.2,30.31 61.14,32.25 71.52,32.25
N$13  (via drill 0.8 pad 1.68)
  Top 0.305: v48.44,22.32 v56.57,30.87
  Bottom 0.305: IC1.10 41.35,25.84 41.35,24.71 44.67,21.39 47.52,21.39 48.68,22.77 v48.44,22.32 | v56.57,30.87 60.46,34.65 J1.6
N$14  (via drill 0.8 pad 1.68)  (2 unrouted)
  Top 0.305: v45.6,22.89 v53.99,30.82
  Bottom 0.305: J1.5 71.36,37.27 70.93,37.27 | IC1.9 42.14,25.5 42.14,24.8 44.16,22.78 45.45,22.78 | v53.99,30.82 60.29,37.12 71.54,37.12 71.5,37.08 71.03,37.08 70.93,36.98 70.89,36.98
N$15
  Bottom 0.305: IC1.2 49.38,29.59 49.58,29.39 50.54,29.39 51.85,30.7 51.85,31.4 52.88,32.43 53.86,32.43 61.16,39.73 J1.4
N$16
  Bottom 0.305: J1.3 61.07,42.27 61.02,42.27 60.81,42.27 58.66,40.12 58.66,38.61 53.68,33.63 52.38,33.63 IC1.1
N$17  (1 unrouted)
  Bottom 0.305: 61.45,44.81 J1.2 | IC1.32 51.32,34.68 53.47,34.68 57.67,38.88 57.67,41.7 60.79,44.82 61.42,44.82
N$18  (1 unrouted)
  Bottom 0.305: TL1.P$2 14.41,50.73 19,50.73 22,47.73 23.27,47.73 | 43.44,50.79 43.5,50.73 | 43.5,50.73 44.55,49.68 44.55,43.93 41.71,41.09 41.71,37.27 42.74,36.24 | 43.5,50.73 35.9,50.73 32.9,47.73 23.5,47.73 23.27,47.73 | R14.2 23.27,47.73
N$19
  Bottom 0.305: J6.1 55.98,46.77 55.98,48.69 55.84,48.83 52.3,48.83 52.3,45.16 49.11,41.97 48.58,41.97 IC1.24
N$20
  Top 0.305: 40.16,73.39 LED5.B
  Top 0.406: IC2.5 35.34,76.33 36.27,75.41 39.38,75.41 40.04,74.75 LED5.B
N$21
  Bottom 0.305: IC1.25 53.53,44.81 J6.2
N$22
  Top 0.406: IC2.4 34.7,78.25 32.64,76.19 LED6.R
N$23
  Bottom 0.305: IC1.26 54.02,44.17 56.46,44.17 60.12,47.83 60.12,49.01 59.63,49.5 51.52,49.5 50.99,48.97 J6.3
N$24
  Top 0.305: R5.2 32.64,69.02 LED6.A
N$25
  Top 0.406: IC2.16 35.34,86.05 35.79,85.6 41.18,85.6 46.46,90.88 J3.2
N$26
  Top 0.406: IC2.17 34.7,85.44 35.42,84.71 41.98,84.71 49,91.73 J3.1
N$27
  Bottom 0.305: IC1.27 54.41,43.43 56.86,43.43 61.18,47.75 61.18,49.5 60.21,50.47 49.38,50.47 48.45,49.54 J6.4
N$28  (1 unrouted)
  Top 0.406: R18.1 50.51,77.61 51.11,77.01 51.11,71.95 50.57,71.41 49.01,71.41
N$29
  Top 0.406: R15.2 44.05,73.27 LED5.A
N$30  (1 unrouted)
  Bottom 0.305: R8.1 42.79,10.87 41.1,12.56 | IC1.13 33.01,20.9 33.01,15.69 36.14,12.56 41.13,12.56
N$31
  Bottom 0.305: IC1.28 54.82,42.71 57.34,42.71 61.95,47.32 61.95,50.36 61.12,51.19 46.88,51.19 45.91,50.22 J6.5
N$33  (1 unrouted)
  Bottom 0.305: IC1.15 31.71,21.86 31.71,15.05 35.33,11.43 37.42,11.43 39.17,9.68 39.17,8.94 39.21,8.94
N$38
  Bottom 0.305: IC1.17 39.36,32.79 38.32,33.83 37.46,33.83 26.8,23.17 26.8,16.82 26.81,14.86 26.81,13.76 28.94,11.64 28.94,7.28 R12.1
N$39  (1 unrouted)
  Bottom 0.305: IC1.16 30.42,21.7 30.42,14.43 33.34,11.51 33.34,10.53 34.89,8.98
N$40
  Bottom 0.305: R9.1 26.93,6.39 26.93,7.35 27.69,8.11 J2.2
N$41
  Bottom 0.305: C8.2 5.4,31.08 5.4,32.23 5.8,32.63 IO1.17
N$45  (2 unrouted)
  Bottom 0.406: 10.1,13.83 11.5,12.43 11.5,10.23 | C1.2 11.47,7.14 C13.2
  Bottom 1.422: USB.P$2 10.1,26.32 10.1,13.83
N$51  (1 unrouted)
  Top 0.406: LED1.+B 54.02,75.46 | R17.2 53.99,75.28
N$53  (1 unrouted)
  Top 0.406: LED2.+B 64.24,74.41 64.24,76.48 62.81,77.91 62.81,78.2
N$54  (1 unrouted)
  Top 0.406: LED2.G 61.23,72.33 61.73,71.83 61.73,68.77 61.08,68.12 60.37,68.12
N$55  (1 unrouted)
  Top 0.406: IC2.3 34.05,79.08 33.78,78.81 32.93,78.81 30.86,76.74
N$58
  Top 0.406: IC2.13 37.3,89.89 36.65,89.89 | 36.65,89.89 IC2.14 | J3.4 41.4,95.51 41.4,97.27 40.82,97.85 38.18,97.85 37.59,97.26 37.59,93.55 36.65,92.61 36.65,89.89
N$59  (1 unrouted)
  Top 0.406: J3.5 38.61,95.28 38.61,89.83 | 38.61,89.83 38.61,87.8 | IC2.12 37.95,89.83 38.61,89.83
N$60
  Top 0.406: IC2.6 36,77.03 36.56,76.47 44.79,76.47 44.98,76.66 47.82,76.66 48.7,75.78 LED1.B
N$61
  Top 0.406: IC2.7 36.65,77.56 36.87,77.34 46.67,77.34 48.53,79.2 54.98,79.2 56.11,78.07 56.11,72 55.54,71.43 53.8,71.43 LED1.+R
N$62  (1 unrouted)
  Top 0.406: 37.98,80.55 37.98,79.19 38.25,78.92 45.46,78.92 47.78,81.24 57.37,81.24 60.51,78.1 60.51,76.27 62.17,74.61 62.17,72.93 62.75,72.35 64.4,72.35 LED2.+G
N$63
  Top 0.305: IC2.8
  Top 0.406: IC2.8 37.31,78.38 37.49,78.2 46.25,78.2 48.06,80.01 56.71,80.01 59.29,77.43 59.29,74.28 LED2.B
RST
  Bottom 0.305: R9.2 28.76,0.76 70.57,0.76 74.18,4.37 74.18,16.83 76.62,19.27 SV2.2
SS  (1 unrouted)
  Bottom 0.305: R8.2 42.78,4.45 43.31,3.92 68.68,3.92 70.77,6.01 70.77,20.59 75.35,25.17 75.35,27.91 76.99,29.55 80.98,29.55
TARGET_SYSTEM_POWER_SUPPLY  (1 unrouted)
V+  (3 unrouted)
  Top 0.406: R19.1 57.42,85.84 56.65,85.07 53.97,85.07 53.94,85.1 52.98,85.1 50.64,82.76 45.96,82.76 45.94,82.74 39.88,82.74 39.26,83.36 32.84,83.36 32.74,83.46 32.74,86.18 | 32.74,86.18 32.74,87.57 | 32.74,86.18 27.1,86.18 26.99,86.29 26.93,86.29 | J4.1 J4.2 J4.3 J4.4 41.46,65.49 41.46,63.41 41.03,62.98 26.32,62.98 25.06,64.24 25.06,85.73 25.66,86.33 26.89,86.33 26.93,86.29 | 26.93,86.29 26.94,86.3 C7.2

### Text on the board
Top: www.prochazka.zde.cz | programmer ATMEL
Bottom: programmer ATMEL | www.prochazka.zde.cz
